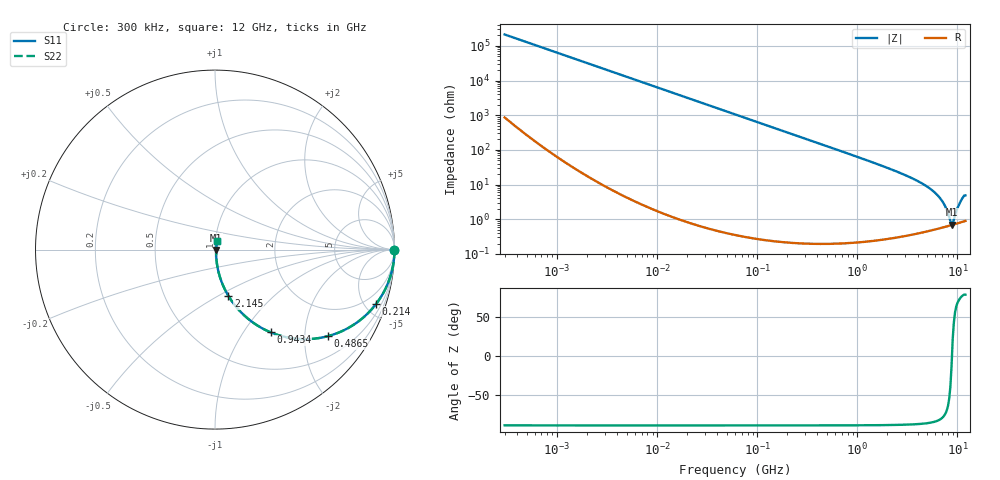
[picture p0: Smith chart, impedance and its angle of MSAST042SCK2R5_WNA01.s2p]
! MSAST042SCK2R5_WNA01  S-PARAMETER MODEL  ( General Type )
! Model Generated by TAIYO YUDEN Corporation (http://www.ty-top.com)
! Version 1.0
! TAIYO YUDEN Control No. 150820
! Copyright(c) 2015 TAIYO YUDEN CO.,LTD. All Rights Reserved.
! Product Description (link to TY-COMPAS)
! https://ds.yuden.co.jp/TYCOMPAS/or/detail?pn=MSAST042SCK2R5AWNA01&u=M
! Products Name : Multilayer Ceramic Capacitors
! Characteristics :
!  Capacitance : 2.5 pF , Rated Voltage : 25V , TCC : CK / C0K
!  Case Size : 0.4 x 0.2 / 0.016 x 0.008 [mm/inch] , Thickness : 0.2 / 0.008 [mm/inch]
!  (Conditions: Temperature = 25 degC , DC Bias Current/Voltage = 0A / 0V)
! External Node Assignments :
!  1  o---| |---o  2
! GND o---------o GND
! Frequency Range : 0.3MHz  -  12000MHz  [ 401 STEP ]
# MHz S RI R 50
! Freq[MHz].  S11 Real  S11 Imag  S21 Real  S21 Imag  S12 Real  S12 Imag  S22 Real  S22 Imag
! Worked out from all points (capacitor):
!   401 points, 300 kHz to 12 GHz, reference 50 ohm
!   read as one part in series: C = 2.49 pF near 316.3 kHz
!   lowest |Z| = 697 mohm at 8.732 GHz (marker M1)
!   series resonance near 8.813 GHz, so ESL is about 130 pH
!   S11 on the Smith chart (normalised r, x): 300 kHz: open; 214 MHz: 1.00, -5.96; 486.5 MHz: 1.00, -2.62; 943.4 MHz: 1.00, -1.34; 2.145 GHz: 1.01, -0.56; 12 GHz: 1.02, +0.10
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0.3  1 -0.00047  2.12e-06 0.00047  2.12e-06 0.00047  1 -0.00047
1.769972  1 -0.00277  9.36e-06 0.00277  9.36e-06 0.00277  1 -0.00277
10.44266  0.9997 -0.0164  0.000272 0.0164  0.000272 0.0164  0.9997 -0.0164
60  0.9912 -0.0932  0.00879 0.0932  0.00879 0.0932  0.9912 -0.0932
213.9924  0.8987 -0.3014  0.1013 0.3014  0.1013 0.3014  0.8987 -0.3014
353.9943  0.764 -0.4241  0.236 0.4241  0.236 0.4241  0.764 -0.4241
486.4723  0.631 -0.4818  0.369 0.4818  0.369 0.4818  0.631 -0.4818
668.5285  0.4741 -0.4983  0.5259 0.4983  0.5259 0.4983  0.4741 -0.4983
943.3804  0.3097 -0.4608  0.6903 0.4608  0.6903 0.4608  0.3097 -0.4608
1403.667  0.1656 -0.369  0.8344 0.369  0.8344 0.369  0.1656 -0.369
2088.533  0.079 -0.265  0.921 0.265  0.921 0.265  0.079 -0.265
2144.601  0.0749 -0.2584  0.9251 0.2584  0.9251 0.2584  0.0749 -0.2584
3841.137  0.0214 -0.1313  0.9786 0.1313  0.9786 0.1313  0.0214 -0.1313
5715.274  0.00902 -0.064  0.991 0.064  0.991 0.064  0.00902 -0.064
7064.448  0.00675 -0.0321  0.9933 0.0321  0.9933 0.0321  0.00675 -0.0321
7648.807  0.0065 -0.0205  0.9935 0.0205  0.9935 0.0205  0.0065 -0.0205
8503.825  0.00664 -0.0053  0.9934 0.0053  0.9934 0.0053  0.00664 -0.0053
8732.115  0.00676 -0.0015  0.9932 0.0015  0.9932 0.0015  0.00676 -0.0015
9207.246  0.0071 0.00666  0.9929 -0.00666  0.9929 -0.00666  0.0071 0.00666
9968.853  0.00791 0.0189  0.9921 -0.0189  0.9921 -0.0189  0.00791 0.0189
10793.46  0.00912 0.0321  0.9909 -0.0321  0.9909 -0.0321  0.00912 0.0321
12000  0.0111 0.047  0.9889 -0.047  0.9889 -0.047  0.0111 0.047
